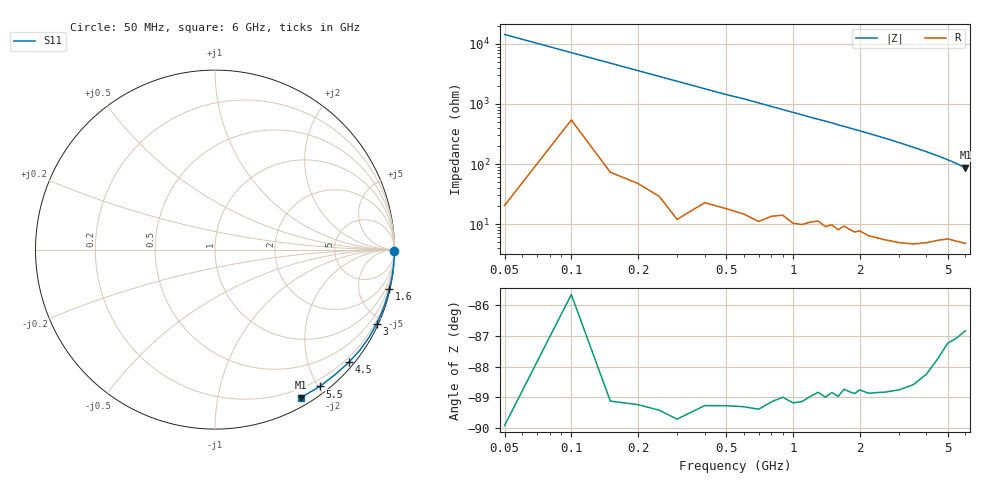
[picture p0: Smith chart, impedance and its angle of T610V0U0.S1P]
! SIEMENS Discrete & RF Semiconductors
! BAT62
! Si Schottky Diode in SOT143
! VR = 10 V
! S-Parameters:  February  1997
# GHz  S  MA  R  50
!  f  S11
! GHz  MAG  ANG
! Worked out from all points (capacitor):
!   34 points, 50 MHz to 6 GHz, reference 50 ohm
!   read as one part to ground: C = 222 fF near 50 MHz
!   lowest |Z| = 86.7 ohm at 6 GHz (marker M1)
!   S11 on the Smith chart (normalised r, x): 50 MHz: open; 1.6 GHz: 0.16, -8.98; 3 GHz: 0.10, -4.57; 4.5 GHz: 0.11, -2.74; 5.5 GHz: 0.10, -2.02; 6 GHz: 0.10, -1.73
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0.05  1 -0.4
0.1  0.9989 -0.8
0.15  0.9997 -1.2
0.3  0.9998 -2.4
0.5  0.9991 -4.0
0.6  0.999 -4.7
0.7  0.999 -5.5
0.8  0.9984 -6.3
1  0.998 -7.9
1.1  0.9977 -8.7
1.3  0.9964 -10.3
1.4  0.9967 -11.0
1.5  0.9959 -11.8
1.6  0.9961 -12.7
1.7  0.9949 -13.5
1.9  0.9949 -15.1
2  0.9941 -15.9
2.2  0.9941 -17.6
2.4  0.9934 -19.3
2.6  0.9927 -21.0
2.8  0.9919 -22.8
3  0.991 -24.7
3.5  0.9879 -29.5
4  0.9828 -34.6
4.5  0.975 -40.1
5  0.9659 -46.0
5.5  0.9601 -52.6
6  0.9533 -59.9
